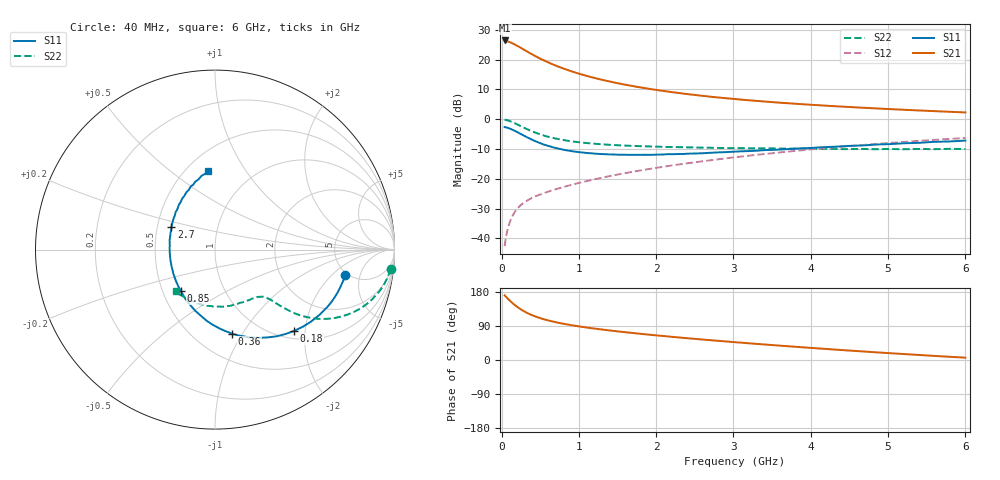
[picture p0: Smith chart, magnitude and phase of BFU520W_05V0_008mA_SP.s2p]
! Filename:  P:\Prog\Test\Noise\ATS_data\Testdata_Net\Run2\BFU520W_APM2013_06_A05_05p0V_008mA_SP_CM01_D.s2p
! Date/Time: Tue 26/Mar/2013 18:01:41
! BFU520W_APM2013_06_A05_05p0V_1to20mA_SP_CM01_Bias5_R.s2p
! MDIF S-parameter v. bias file
! BFU520W_APM2013_06_A05_05p0V_1to20mA_SP_CM01
! Date/time Thu Mar 21 14:22:37 2013
! VAR V_out= 5.0000
! VAR I_out= 8.0000
! VAR V_in= 0.8370
! VAR I_in= 0.0905
! Device data file deembeded for feedlines and parallel
! Original file: \Run2\BFU520W_APM2013_06_A05_05p0V_008mA_SP_CM01_R.s2p
! Feed-files: PR019V01_070313_Feed1.s2p, PR019V01_070313_Feed2.s2p
! Parallel-file: PR019V01_070313_Par.s2p
# MHz S MA R 50
!  Freq-MHz  S11-mag  S11-arg  S21-mag  S21-arg  S12-mag  S12-arg  S22-mag  S22-arg
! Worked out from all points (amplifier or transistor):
!   98 points, 40 MHz to 6 GHz, reference 50 ohm
!   highest |S21| = 26.5 dB at 40 MHz (marker M1)
!   |S21| within 3 dB of that: start of sweep to 283.4 MHz
!   unconditionally stable (mu >= 1): 1.533 GHz to 2.762 GHz
!   at 300 MHz: K = 0.45, MSG = 25.5 dB, |S12| = -27.8 dB
!   at 1.6 GHz: K = 1.00, MAG = 14.5 dB, |S12| = -18.1 dB
!   at 6 GHz: K = 0.87, MSG = 4.3 dB, |S12| = -6.3 dB
!   S11 on the Smith chart (normalised r, x): 40 MHz: 4.75, -2.96; 180 MHz: 1.16, -1.75; 360 MHz: 0.74, -0.90; 850 MHz: 0.62, -0.31; 2.7 GHz: 0.59, +0.16; 6 GHz: 0.64, +0.69
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40  0.7388 -11.0  21.03 170.7  0.007396 83.9  0.9843 -6.3
50  0.7349 -13.7  21.01 168.5  0.009137 82.9  0.9795 -7.8
80  0.7177 -21.8  20.32 162.1  0.01431 79.4  0.9579 -12.3
120  0.6862 -32.0  19.44 154.2  0.02061 75.0  0.9182 -17.6
140  0.669 -36.8  18.89 150.5  0.02347 73.0  0.8951 -20.0
180  0.6316 -45.9  17.71 143.8  0.02872 69.6  0.847 -24.3
220  0.5935 -54.4  16.65 137.7  0.0332 67.1  0.799 -27.7
260  0.5564 -61.9  15.53 132.3  0.03711 65.0  0.7533 -30.6
320  0.5056 -72.5  14 125.4  0.04227 62.8  0.6913 -33.9
360  0.477 -78.7  13.05 121.5  0.04527 61.9  0.6552 -35.5
440  0.4272 -89.7  11.45 114.7  0.0508 60.9  0.5948 -37.8
550  0.3745 -102.7  9.709 107.4  0.05757 60.7  0.5312 -39.6
700  0.3296 -117.3  7.974 99.8  0.06671 61.3  0.4746 -40.9
850  0.2996 -129.6  6.742 93.8  0.0758 62.2  0.437 -41.6
1050  0.2761 -143.2  5.584 87.3  0.08824 63.5  0.4045 -42.6
1500  0.2544 -167.3  4.035 75.6  0.1177 64.8  0.3666 -45.8
2050  0.255 171.5  3.041 64.1  0.1562 64.7  0.3457 -51.7
2700  0.2735 152.6  2.393 52.3  0.2045 62.7  0.3323 -61.5
3100  0.2892 142.7  2.136 45.7  0.2363 60.8  0.3273 -68.0
4100  0.3362 123.4  1.721 30.5  0.32 54.5  0.3173 -87.7
5200  0.3948 106.0  1.444 15.7  0.4162 45.3  0.3136 -112.6
6000  0.4385 95.1  1.302 6.2  0.4843 37.7  0.3162 -132.9
